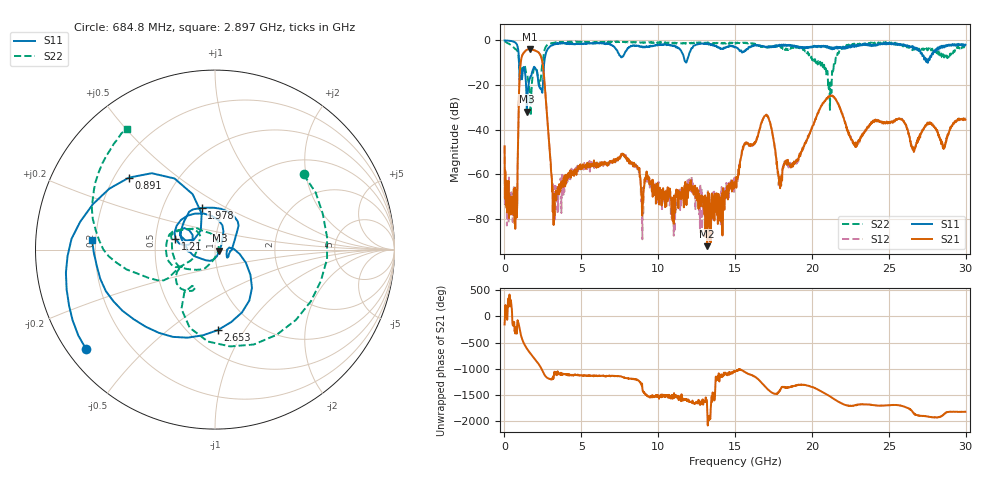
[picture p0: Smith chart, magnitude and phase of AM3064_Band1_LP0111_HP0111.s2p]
# Hz S DB R 50.0
!freq dBS11 angS11 dBS21 angS21 dBS12 angS12 dBS22 angS22
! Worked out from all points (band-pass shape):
!   1600 points, 10 MHz to 29.98 GHz, reference 50 ohm
!   highest |S21| = -3.88 dB at 1.678 GHz (marker M1); lowest = -92.2 dB at 13.19 GHz (marker M2)
!   |S21| within 3 dB of the highest: 1.149 GHz to 2.356 GHz (1.207 GHz wide, 68.9 % of centre)
!   lowest |S11| = -31.9 dB at 1.453 GHz (marker M3), VSWR 1.05, Z = 52.5 - j0.615 ohm
!   |S11| at or under -10 dB: 949.4 MHz to 2.586 GHz (1.637 GHz wide, 92.6 % of centre); 27.52451 GHz to 27.54471 GHz (20.2 MHz wide, 0.0734 % of centre)
!   |S22| runs from -33.8 to -0.4 dB; largest |S21 - S12| = 0.0076
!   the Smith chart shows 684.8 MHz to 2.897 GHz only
!   S11 on the Smith chart (normalised r, x): 684.8 MHz: 0.05, -0.34; 891 MHz: 0.26, +0.34; 1.21 GHz: 0.63, +0.08; 1.978 GHz: 0.78, +0.38; 2.653 GHz: 0.68, -0.77; 2.897 GHz: 0.19, +0.04
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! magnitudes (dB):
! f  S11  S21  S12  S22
! 10 MHz  0.0  -47.5  -47.5  -0.4
! 684.8 MHz  -0.8  -66.1  -71.1  -3.8
! 891 MHz  -4.1  -42.2  -42.5  -5.8
! 1.21 GHz  -12.8  -6.0  -6.0  -11.8
! 1.453 GHz  -31.9  -4.2  -4.2  -15.7
! 1.678 GHz  -16.4  -3.9  -3.9  -29.7
! 1.978 GHz  -12.3  -4.5  -4.5  -12.4
! 2.653 GHz  -7.0  -22.8  -22.8  -3.4
! 2.897 GHz  -3.3  -44.9  -44.8  -1.6
! 3.346 GHz  -1.6  -67.4  -68.4  -1.0
! 5.015 GHz  -1.4  -57.1  -57.3  -0.7
! 10 GHz  -2.1  -67.3  -68.7  -1.0
! 13.19 GHz  -1.5  -92.2  -72.7  -1.1
! 15 GHz  -3.0  -63.9  -65.0  -1.4
! 16.95 GHz  -2.8  -33.8  -33.7  -2.9
! 17.91 GHz  -2.0  -62.3  -62.4  -3.0
! 19.99 GHz  -3.2  -39.4  -39.4  -8.2
! 21.21 GHz  -3.7  -24.8  -24.6  -18.8
! 22.8 GHz  -2.2  -46.5  -46.3  -2.0
! 25 GHz  -1.2  -36.9  -36.2  -1.1
! 26.61 GHz  -3.8  -48.6  -49.3  -3.3
! 29.98 GHz  -1.9  -35.6  -35.3  -2.9
